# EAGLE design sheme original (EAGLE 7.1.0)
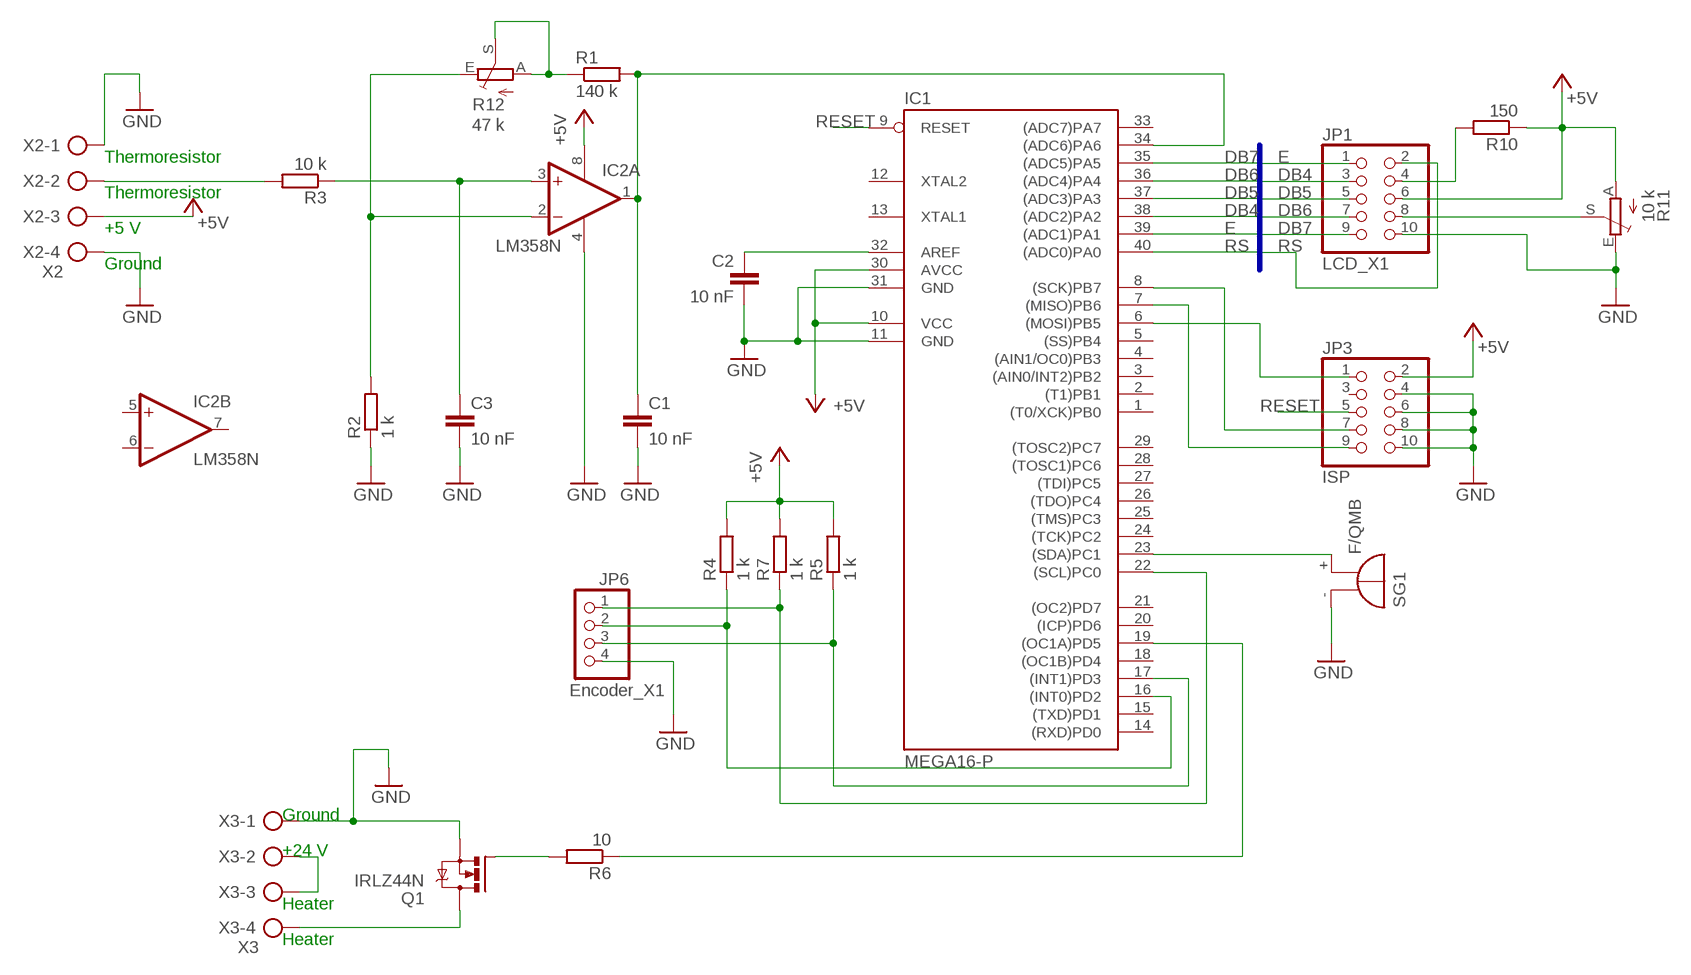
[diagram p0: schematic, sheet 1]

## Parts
C1  10 nF  C-EU050-024X044  [C050-024X044]
C2  10 nF  C-EU050-024X044  [C050-024X044]
C3  10 nF  C-EU050-024X044  [C050-024X044]
IC1  MEGA16-P  [DIL40]
IC2  LM358N  [DIL08]
JP1  LCD_X1  PINHD-2X5  [2X05]
JP3  ISP  PINHD-2X5  [2X05]
JP6  Encoder_X1  PINHD-1X4  [1X04]
Q1  IRLZ44N  IRLZ44Z  [TO220BH]
R1  140 k  R-EU_0207/10  [0207/10]
R2  1 k  R-EU_0207/10  [0207/10]
R3  10 k  R-EU_0207/10  [0207/10]
R4  1 k  R-EU_0207/10  [0207/10]
R5  1 k  R-EU_0207/10  [0207/10]
R6  10  R-EU_0207/10  [0207/10]
R7  1 k  R-EU_0207/10  [0207/10]
R10  150  R-EU_0207/10  [0207/10]
R11  10 k  TRIM_EU-RJ6  [RJ6]
R12  47 k  TRIM_EU-RJ6  [RJ6]
SG1  F/QMB  [F/QMB]
X2  X2  AK500/4  [AK500/4]
X3  X3  AK500/4  [AK500/4]

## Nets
+5V: IC1.10(VCC) IC1.30(AVCC) IC2.8(P:V+) JP1.6 JP3.2 R4.2 R5.2 R7.2 R10.1 R11.A X2.3
DB4: IC1.38((ADC2)PA2) JP1.3
DB5: IC1.37((ADC3)PA3) JP1.5
DB6: IC1.36((ADC4)PA4) JP1.7
DB7: IC1.35((ADC5)PA5) JP1.9
E: IC1.39((ADC1)PA1) JP1.1
GND: C1.2 C2.2 C3.2 IC1.11(GND) IC1.31(GND) IC2.4(P:V-) JP1.10 JP3.4 JP3.6 JP3.8 JP3.10 JP6.4 Q1.S R2.1 R11.E SG1.-(+) X2.1 X2.4 X3.1
N$1: IC1.23((SDA)PC1) SG1.+(-)
N$2: C2.1 IC1.32(AREF)
N$11: JP1.4 R10.2
N$12: IC1.6((MOSI)PB5) JP3.1
N$13: JP1.8 R11.S
N$14: IC1.7((MISO)PB6) JP3.9
N$15: IC1.8((SCK)PB7) JP3.7
N$17: IC1.17((INT1)PD3) JP6.3 R5.1
N$18: IC1.22((SCL)PC0) JP6.1 R7.1
N$19: IC1.16((INT0)PD2) JP6.2 R4.1
N$20: C1.1 IC1.34((ADC6)PA6) IC2.1(A:OUT) R1.2
N$21: R1.1 R12.A R12.S
N$22: C3.1 IC2.3(A:+IN) R3.1
N$23: IC2.2(A:-IN) R2.2 R12.E
N$24: IC1.19((OC1A)PD5) R6.1
N$25: Q1.G R6.2
N$26: X3.2 X3.3
N$27: R3.2 X2.2
N$28: Q1.D X3.4
RESET: IC1.9(RESET) JP3.5
RS: IC1.40((ADC0)PA0) JP1.2
Unconnected: IC1.1((T0/XCK)PB0) IC1.2((T1)PB1) IC1.3((AIN0/INT2)PB2) IC1.4((AIN1/OC0)PB3) IC1.5((SS)PB4) IC1.12(XTAL2) IC1.13(XTAL1) IC1.14((RXD)PD0) IC1.15((TXD)PD1) IC1.18((OC1B)PD4) IC1.20((ICP)PD6) IC1.21((OC2)PD7) IC1.24((TCK)PC2) IC1.25((TMS)PC3) IC1.26((TDO)PC4) IC1.27((TDI)PC5) IC1.28((TOSC1)PC6) IC1.29((TOSC2)PC7) IC1.33((ADC7)PA7) IC2.5(B:+IN) IC2.6(B:-IN) IC2.7(B:OUT) JP3.3

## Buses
E,DB4,DB5,DB6,DB7,RS

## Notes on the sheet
- Thermoresistor
- Thermoresistor
- +5 V
- Ground
- Ground
- +24 V
- Heater
- Heater

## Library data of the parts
C1-C3 = rcl:C-EU: CAPACITOR, European symbol
IC1 = atmel:MEGA16-P: MICROCONTROLLER 16 Kbytes FLASH 1 kbytes SRAM 512 bytes EEPROM USART 8-channel 10 bit ADC Source: avr.lbr; MPN: ATMEGA16-16PU; OC_FARNELL: 9171142; OC_NEWARK: 01M6885
IC2 = linear:LM358: OP AMP also LM158; LM258; LM2904 Source: http://cache.national.com/ds/LM/LM158.pdf
JP1 JP3 = pinhead:PINHD-2X5: PIN HEADER
JP6 = pinhead:PINHD-1X4: PIN HEADER
Q1 = transistor-power:IRLZ44Z: N-Channel HEXFET® Power MOSFET Logic Level AUTOMOTIVE MOSFET Source: http://www.irf.com/product-info/datasheets/data/irlz44zpbf.pdf
R1-R7 R10 = rcl:R-EU_: RESISTOR, European symbol
R11 R12 = pot:TRIM_EU-: POTENTIOMETER
SG1 = buzzer:F/QMB: BUZZER; OC_FARNELL: unknown; OC_NEWARK: unknown
X2 X3 = con-ptr500:AK500/4: CONNECTOR; OC_FARNELL: unknown; OC_NEWARK: unknown

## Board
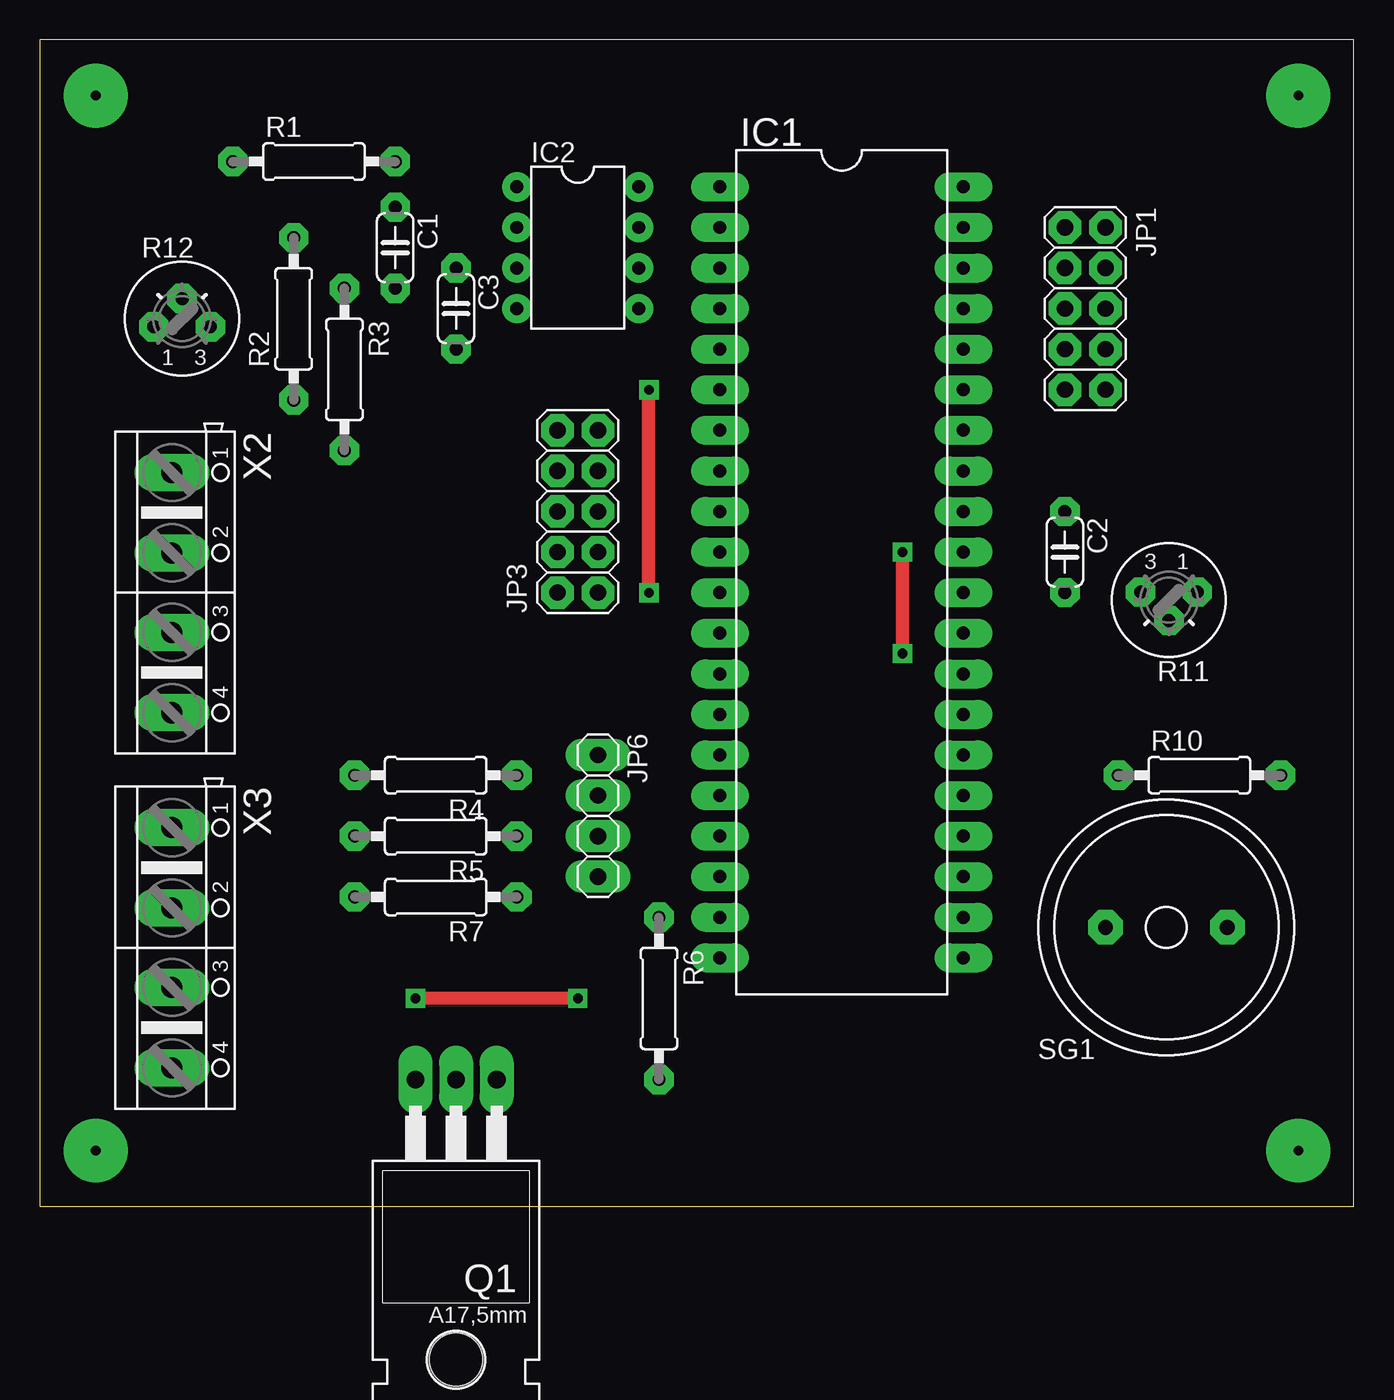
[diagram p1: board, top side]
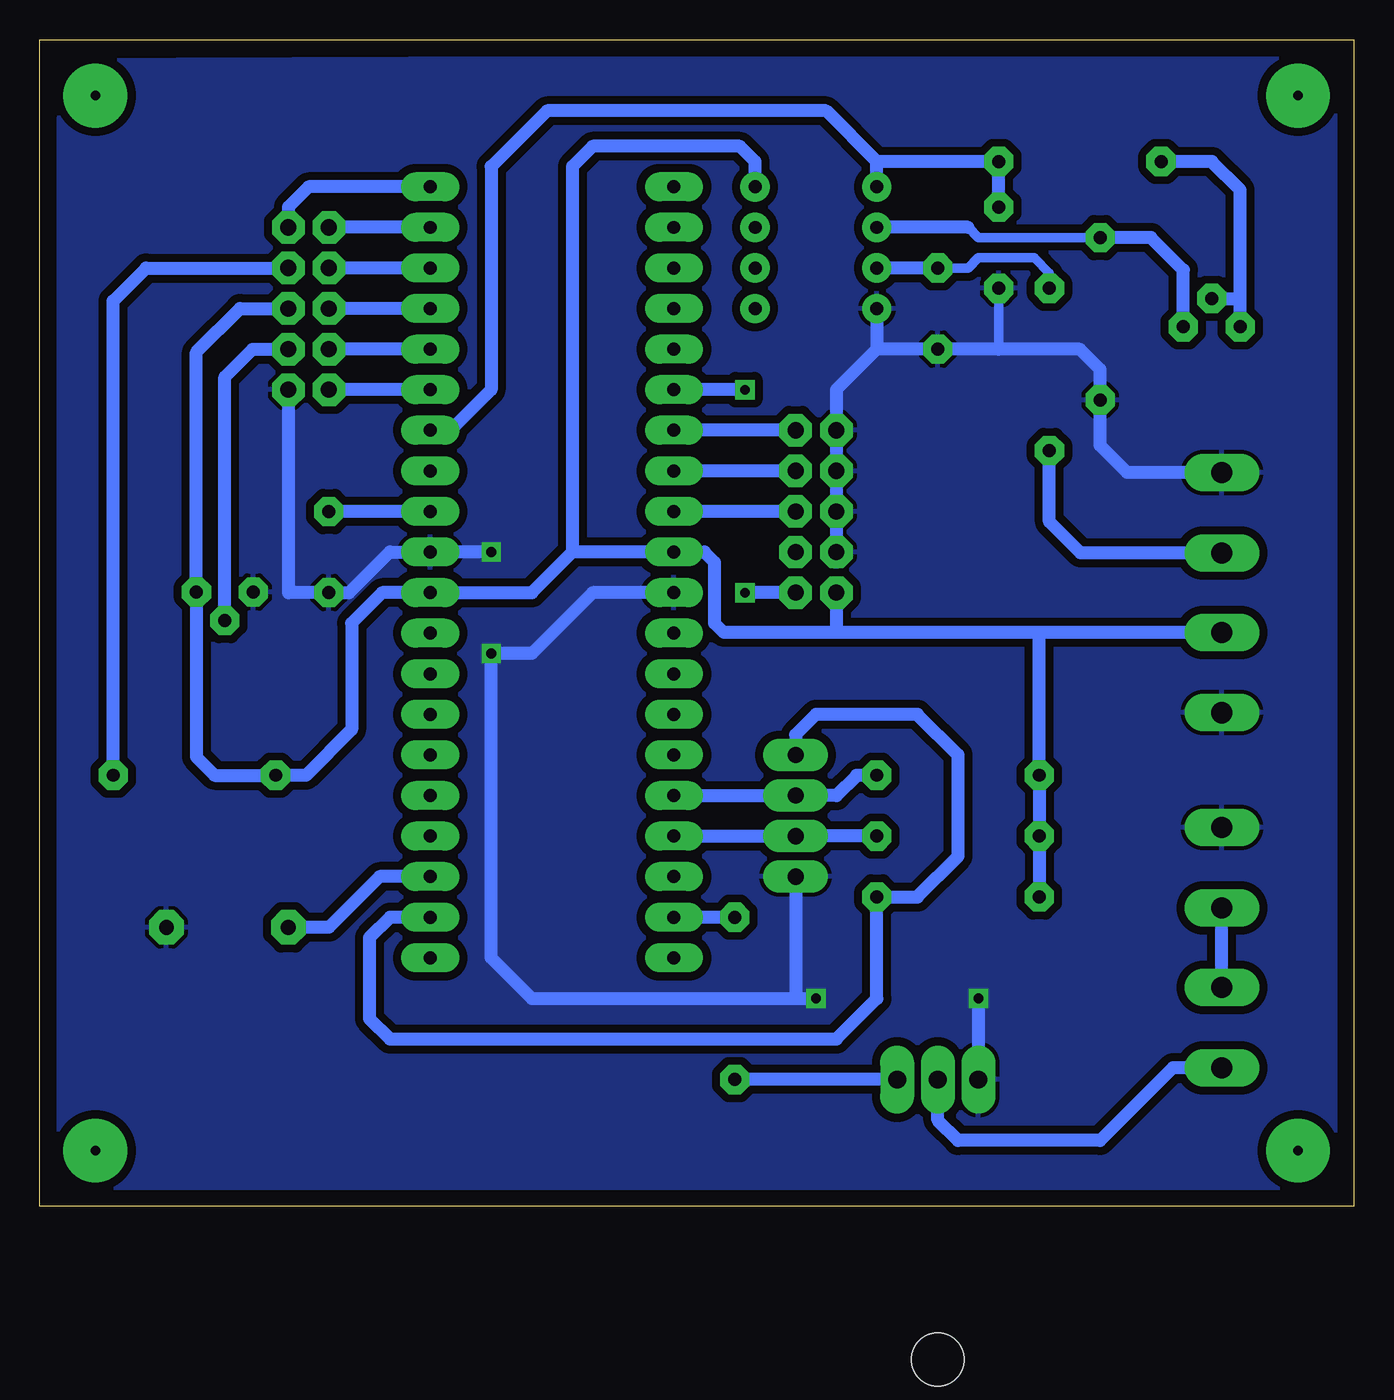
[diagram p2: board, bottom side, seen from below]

Size 82.21 x 73.01 mm. Coordinates in mm from the lower left corner, seen from the top.
Outline: 0,0 82.21,0 82.21,73.01 0,73.01 0,0
Copper layers (1*16): Top 0.035mm / dielectric 1.5mm / Bottom 0.035mm
Design rules "default *": minimum track width 0.3mm, minimum drill 20mil, track to track 20mil, track to pad 12mil, pad to pad 12mil, via to via 12mil, smd to smd 8mil, copper to edge 40mil, drill to drill 20mil, minimum pad ring 20mil, minimum via ring 12mil, stop-mask expansion 4mil, vias tented up to drill 0mil, thermal gap 10mil

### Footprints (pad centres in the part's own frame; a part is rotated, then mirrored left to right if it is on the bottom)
C050-024X044 = drill 0.813 octagon: 1 -2.54,0; 2 2.54,0
DIL40 = drill 0.813 long: 1 -24.13,-7.62; 2 -21.59,-7.62; 3 -19.05,-7.62; 4 -16.51,-7.62; 5 -13.97,-7.62; 6 -11.43,-7.62; 7 -8.89,-7.62; 8 -6.35,-7.62; 9 -3.81,-7.62; 10 -1.27,-7.62; 11 1.27,-7.62; 12 3.81,-7.62; 13 6.35,-7.62; 14 8.89,-7.62; 15 11.43,-7.62; 16 13.97,-7.62; 17 16.51,-7.62; 18 19.05,-7.62; 19 21.59,-7.62; 20 24.13,-7.62; 21 24.13,7.62; 22 21.59,7.62; 23 19.05,7.62; 24 16.51,7.62; 25 13.97,7.62; 26 11.43,7.62; 27 8.89,7.62; 28 6.35,7.62; 29 3.81,7.62; 30 1.27,7.62; 31 -1.27,7.62; 32 -3.81,7.62; 33 -6.35,7.62; 34 -8.89,7.62; 35 -11.43,7.62; 36 -13.97,7.62; 37 -16.51,7.62; 38 -19.05,7.62; 39 -21.59,7.62; 40 -24.13,7.62
DIL08 = drill 0.813 pad 1.27: 1 -3.81,-3.81; 2 -1.27,-3.81; 3 1.27,-3.81; 4 3.81,-3.81; 5 3.81,3.81; 6 1.27,3.81; 7 -1.27,3.81; 8 -3.81,3.81
2X05 = drill 1.016 octagon: 1 -5.08,-1.27; 2 -5.08,1.27; 3 -2.54,-1.27; 4 -2.54,1.27; 5 0,-1.27; 6 0,1.27; 7 2.54,-1.27; 8 2.54,1.27; 9 5.08,-1.27; 10 5.08,1.27
1X04 = drill 1.016 long: 1 -3.81,0; 2 -1.27,0; 3 1.27,0; 4 3.81,0
TO220BH = drill 1.118 long: D 0,-6.35; G -2.54,-6.35; S 2.54,-6.35 | hole 3.302: 0,11.176
0207/10 = drill 0.813 octagon: 1 -5.08,0; 2 5.08,0
RJ6 = drill 0.813 octagon: A -1.778,-0.508; E 1.778,-0.508; S 0,1.27
F/QMB = drill 0.914 pad 2.159 octagon: + 3.81,0; - -3.81,0
AK500/4 = drill 1.321 long: 1 -7.518,0; 2 -2.489,0; 3 2.489,0; 4 7.518,0

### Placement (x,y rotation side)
C1  22.22,60.01 270 top
C2  64.14,40.96 270 top
C3  26.03,56.2 270 top
IC1  50.16,39.69 270 top
IC2  33.66,60.01 270 top
JP1  65.41,56.2 270 top
JP3  33.66,43.5 90 top
JP6  34.92,24.45 270 top
Q1  26.03,1.59 180 top
R1  17.14,65.41 0 top
R2  15.88,55.56 90 top
R3  19.05,52.39 270 top
R4  24.77,26.99 180 top
R5  24.77,23.18 180 top
R6  38.73,13.02 270 top
R7  24.77,19.37 180 top
R10  72.55,26.99 0 top
R11  70.64,37.94 180 top
R12  8.89,55.56 0 top
SG1  70.48,17.46 180 top
X2  8.25,38.42 270 top
X3  8.25,16.19 270 top

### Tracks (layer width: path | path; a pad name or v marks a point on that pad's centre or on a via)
+5V
  Bottom 0.813: 48.89,40.96 51.44,38.42 IC1.30 60.8,38.42 62.71,36.51 62.71,29.84 65.56,26.99 R10.1 71.28,26.99 72.42,28.13 R11.A 72.42,53.47 69.69,56.2 JP1.6 | IC2.8 37.47,65.41 38.42,66.36 47.62,66.36 48.89,65.09 48.89,40.96 | R7.2 R5.2 R4.2 19.68,35.93 | X2.3 19.68,35.93 | 19.68,35.93 32.39,35.93 | 32.39,35.93 39.42,35.93 40,36.51 40,40.32 40.64,40.96 IC1.10 48.89,40.96 | JP3.2 32.39,35.93
DB4
  Bottom 0.813: IC1.38 JP1.3
DB5
  Bottom 0.813: IC1.37 JP1.5
DB6
  Bottom 0.813: IC1.36 JP1.7
DB7
  Bottom 0.813: IC1.35 JP1.9
E
  Bottom 0.813: IC1.39 JP1.1
GND  (via drill 0.6)
  Top 0.813: v53.97,34.61 v53.97,40.96 | v33.66,13.02 v23.5,13.02
  Bottom 0.61: C1.2 22.22,53.66
  Bottom 0.813: IC1.11 47.62,38.42 51.44,34.61 v53.97,34.61 53.97,15.56 51.44,13.02 34.92,13.02 | v53.97,40.96 IC1.31 60.33,40.96 62.86,38.42 C2.2 66.67,38.42 JP1.10 | JP3.4 JP3.6 JP3.8 JP3.10 32.39,51.12 29.84,53.66 | 34.92,13.02 v33.66,13.02 | v23.5,13.02 Q1.S | JP6.4 34.92,13.02 | X2.1 14.19,45.94 15.88,47.63 R2.1 15.88,52.39 17.14,53.66 22.22,53.66 C3.2 29.84,53.66 | IC2.4 29.84,53.66
  pour Bottom: 0.95,72.07 0.95,0.95 81.28,0.95 80.96,71.75
N$1
  Bottom 0.813: IC1.23 60.96,20.64 64.14,17.46 SG1.+
N$2
  Bottom 0.813: IC1.32 C2.1
N$3  (via drill 0.6 pad 4)
  other vias: 78.74,69.53
N$4  (via drill 0.6 pad 4)
  other vias: 3.49,69.53
N$5  (via drill 0.6 pad 4)
  other vias: 78.74,3.49
N$6  (via drill 0.6 pad 4)
  other vias: 3.49,3.49
N$11
  Bottom 0.813: R10.2 77.63,56.67 75.56,58.74 JP1.4
N$12  (via drill 0.6)
  Top 0.813: v38.1,38.42 v38.1,51.12
  Bottom 0.813: JP3.1 v38.1,38.42 | v38.1,51.12 IC1.6
N$13
  Bottom 0.813: R11.S 70.64,51.91 68.9,53.66 JP1.8
N$14
  Bottom 0.813: JP3.9 IC1.7
N$15
  Bottom 0.813: JP3.7 IC1.8
N$17
  Bottom 0.813: IC1.17 JP6.3 R5.1
N$18
  Bottom 0.813: JP6.1 34.92,29.53 33.66,30.8 27.3,30.8 24.77,28.26 24.77,21.91 27.3,19.37 R7.1 29.84,13.02 32.39,10.48 60.33,10.48 61.59,11.75 61.59,16.83 60.33,18.1 IC1.22
N$19
  Bottom 0.813: IC1.16 JP6.2 32.39,25.72 31.11,26.99 R4.1
N$20
  Bottom 0.813: IC2.1 29.84,65.41 | 29.84,65.41 33.02,68.58 50.48,68.58 53.97,65.09 53.97,51.12 56.52,48.58 IC1.34 | C1.1 R1.2 29.84,65.41
N$21
  Bottom 0.813: R12.A 7.11,56.83 | 7.11,56.83 7.11,63.63 8.89,65.41 R1.1 | R12.S 7.11,56.83
N$22
  Bottom 0.61: C3.1 24.13,58.74 23.5,59.37 20,59.37 19.05,58.42 R3.1
  Bottom 0.813: C3.1 IC2.3
N$23
  Bottom 0.61: 24.13,61.28 23.5,60.64 R2.2
  Bottom 0.813: 24.13,61.28 IC2.2 | R12.E 10.67,58.61 12.7,60.64 R2.2
N$24
  Bottom 0.813: R6.1 IC1.19
N$25
  Bottom 0.813: Q1.G R6.2
N$26
  Bottom 0.813: X3.3 X3.2
N$27
  Bottom 0.813: X2.2 17.09,40.91 19.05,42.86 R3.2
N$28
  Bottom 0.813: X3.4 11.33,8.67 15.88,4.13 24.77,4.13 26.03,5.4 Q1.D
RESET
  Bottom 0.813: JP3.5 IC1.9
RS
  Bottom 0.813: IC1.40 65.41,63.82 66.67,62.55 JP1.2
